TYPE STR_HEATER_LINE_SYS_IN :
STRUCT
	PV	:	REAL	;
	Temp_Hi_Alarm	:	UINT	;
	Working_Output	:	REAL	;
	Working_SP	:	REAL	;
	Inhibit_state	:	BIT	;
	TC_Error	:	BIT	;
	Auto_Manual	:	BIT	;
	

END_STRUCT
END_TYPE
